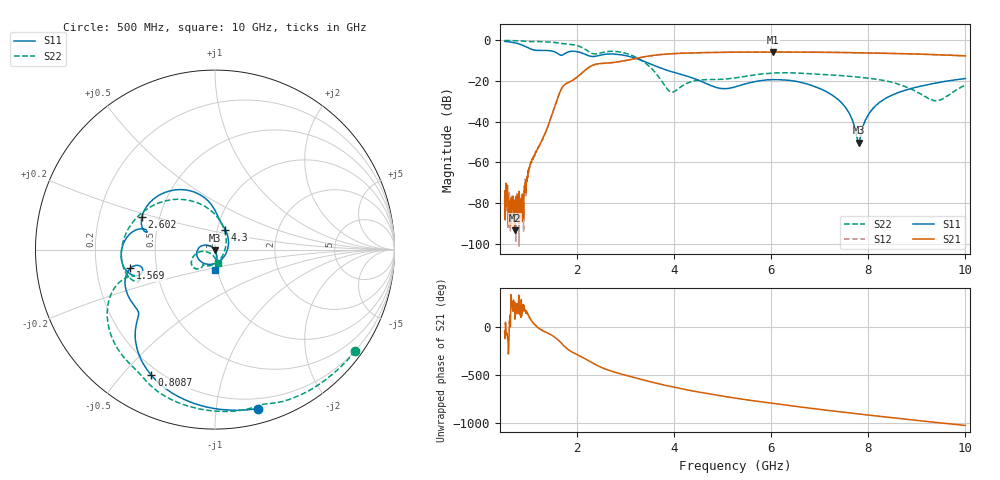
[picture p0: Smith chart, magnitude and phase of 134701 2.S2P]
!  2-Port S-parameters saved by WinCal
! VAR MeasName=S-Parameters (CALIBRATED_DATA) read from VNA (N5242A)
! VAR MeasDate=2013-7-3 16:19:29
! VAR NAME=134701 2
! VAR FILENAME=134701 2.S2P
! VAR DATE=2013-7-3 16:19:29
! VAR PHYS_PORTS=1,2
# Hz S MA R 50
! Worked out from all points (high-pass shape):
!   1601 points, 500 MHz to 10 GHz, reference 50 ohm
!   highest |S21| = -6.01 dB at 6.04 GHz (marker M1); lowest = -93.2 dB at 713.8 MHz (marker M2)
!   |S21| within 3 dB of the highest: 3.229 GHz to end of sweep
!   lowest |S11| = -50.3 dB at 7.809 GHz (marker M3), VSWR 1.01, Z = 49.8 - j0.224 ohm
!   |S11| at or under -10 dB: 3.315 GHz to end of sweep
!   |S22| runs from -29.8 to -0.3 dB; largest |S21 - S12| = 0.0023
!   S11 on the Smith chart (normalised r, x): 500 MHz: 0.12, -1.30; 808.8 MHz: 0.17, -0.60; 1.569 GHz: 0.35, -0.10; 2.602 GHz: 0.40, +0.18; 4.3 GHz: 1.09, +0.25; 10 GHz: 0.98, -0.22
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5e8  0.9177 -74.9  0.0001101 -41.5  0.0001776 -122.6  0.963 -35.9
7.1375e8  0.843 -104.3  2.197e-05 79.9  8.396e-05 -88.6  0.9499 -51.1
8.0875e8  0.785 -116.8  0.0001221 158.0  9.108e-05 78.2  0.9418 -57.9
8.91875e8  0.7164 -126.6  4.266e-05 -161.0  2.018e-05 -152.7  0.9315 -63.9
1.04625e9  0.5889 -137.5  0.001045 68.6  0.00106 70.9  0.9023 -73.7
1.56875e9  0.4825 -167.6  0.03103 -121.0  0.03084 -120.8  0.8501 -112.5
1.717188e9  0.4364 -161.7  0.07579 165.5  0.07539 165.3  0.803 -122.9
2.085312e9  0.479 169.1  0.1512 48.1  0.1505 48.0  0.6559 -154.4
2.601875e9  0.4458 156.1  0.2692 -83.2  0.2684 -83.2  0.5131 -165.1
3.177812e9  0.3597 113.8  0.3446 -168.4  0.3439 -168.3  0.3901 136.2
3.670625e9  0.2144 89.3  0.43 128.4  0.4294 128.5  0.1272 66.9
3.937812e9  0.1665 81.3  0.4555 97.4  0.4553 97.5  0.05259 -18.6
4.3e9  0.1247 62.8  0.4747 60.1  0.4748 60.2  0.09052 -103.0
5.25e9  0.07059 -74.3  0.4977 -21.1  0.4979 -21.1  0.1162 -127.0
6.039688e9  0.1061 -152.1  0.5009 -77.6  0.4995 -77.6  0.1537 -137.6
6.835312e9  0.07598 163.5  0.4974 -128.9  0.4971 -128.9  0.1471 -153.1
7.470625e9  0.02682 142.3  0.4879 -167.2  0.4889 -167.2  0.1322 -160.0
7.809062e9  0.003048 -132.4  0.4823 173.1  0.4816 173.1  0.1218 -163.8
8.040625e9  0.01745 -73.9  0.4769 159.8  0.4768 159.9  0.1131 -166.0
8.420625e9  0.0406 -75.1  0.4672 138.5  0.4665 138.5  0.09605 -170.7
9.388438e9  0.08775 -83.9  0.4321 85.9  0.4327 85.9  0.03253 -128.1
1e10  0.113 -89.2  0.4043 54.0  0.4046 54.0  0.07846 -79.6
